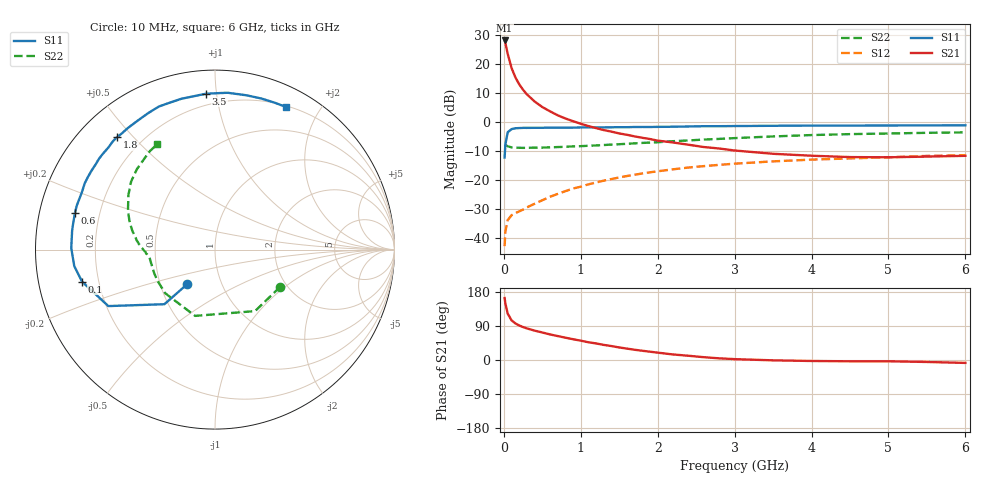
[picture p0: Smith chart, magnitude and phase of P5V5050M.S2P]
! SIEMENS Small Signal Semiconductors
! BFP183
! Si NPN RF Bipolar Junction Transistor in SOT143
! VCE = 0.5 V  IC = 50 mA
! Common Emitter S-Parameters:  March  1996
# GHz  S  MA  R  50
!  f  S11  S21  S12  S22
! GHz  MAG  ANG  MAG  ANG  MAG  ANG  MAG  ANG
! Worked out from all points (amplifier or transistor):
!   36 points, 10 MHz to 6 GHz, reference 50 ohm
!   highest |S21| = 28.2 dB at 10 MHz (marker M1)
!   |S21| within 3 dB of that: start of sweep to 37.03 MHz
!   unconditionally stable (mu >= 1): start of sweep to 30.48 MHz; 121.3 MHz to end of sweep
!   at 250 MHz: K = 1.53, MAG = 16.4 dB, |S12| = -30.1 dB
!   at 1.4 GHz: K = 2.12, MAG = 2.2 dB, |S12| = -19.6 dB
!   at 6 GHz: K = 1.44, MAG = -4.0 dB, |S12| = -11.4 dB
!   S11 on the Smith chart (normalised r, x): 10 MHz: 0.69, -0.28; 100 MHz: 0.14, -0.12; 600 MHz: 0.11, +0.13; 1.8 GHz: 0.11, +0.45; 3.5 GHz: 0.13, +0.94; 6 GHz: 0.21, +1.60
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0.01  0.2468 -128.8  25.77 163.6  0.0073 59.7  0.4181 -29.9
0.02  0.4146 -132.8  23.21 149.3  0.0131 54.3  0.4089 -56.9
0.05  0.6726 -152.1  15.19 122.4  0.0205 41.0  0.3856 -106.7
0.1  0.7621 -166.5  8.666 104.7  0.025 32.6  0.3689 -138.8
0.15  0.7894 -173.3  5.957 96.5  0.0271 33.9  0.3646 -152.1
0.2  0.7945 -177.4  4.515 91.1  0.0291 36.9  0.3633 -158.9
0.25  0.8008 179.4  3.633 86.9  0.0312 39.3  0.362 -163.0
0.3  0.8004 176.8  3.032 83.4  0.0341 42.9  0.3627 -165.8
0.4  0.803 172.4  2.283 77.5  0.0393 47.8  0.365 -169.5
0.5  0.8039 169.1  1.832 72.6  0.0452 50.7  0.366 -171.7
0.6  0.8064 165.5  1.545 67.5  0.0519 53.0  0.3697 -173.4
0.7  0.8082 162.3  1.32 63.2  0.0582 54.6  0.3738 -174.7
0.8  0.8069 159.0  1.163 58.9  0.0649 54.9  0.3781 -175.8
1.1  0.8155 150.4  0.86 46.8  0.085 54.8  0.3936 -178.9
1.5  0.8218 139.4  0.642 33.1  0.1119 51.6  0.4185 176.7
1.8  0.8306 131.1  0.54 24.4  0.1309 48.3  0.4407 173.1
2.2  0.8378 120.9  0.448 14.6  0.1546 42.8  0.4719 167.3
2.6  0.8564 111.4  0.374 7.4  0.1754 37.3  0.5033 161.3
3.5  0.87 93.3  0.286 -0.9  0.2118 25.2  0.5698 147.9
4.5  0.8775 78.4  0.251 -3.4  0.2381 13.3  0.6249 134.1
5.5  0.8834 67.9  0.256 -5.2  0.263 3.5  0.6581 123.4
6  0.8876 63.5  0.264 -7.7  0.2705 -1.5  0.6698 118.6
